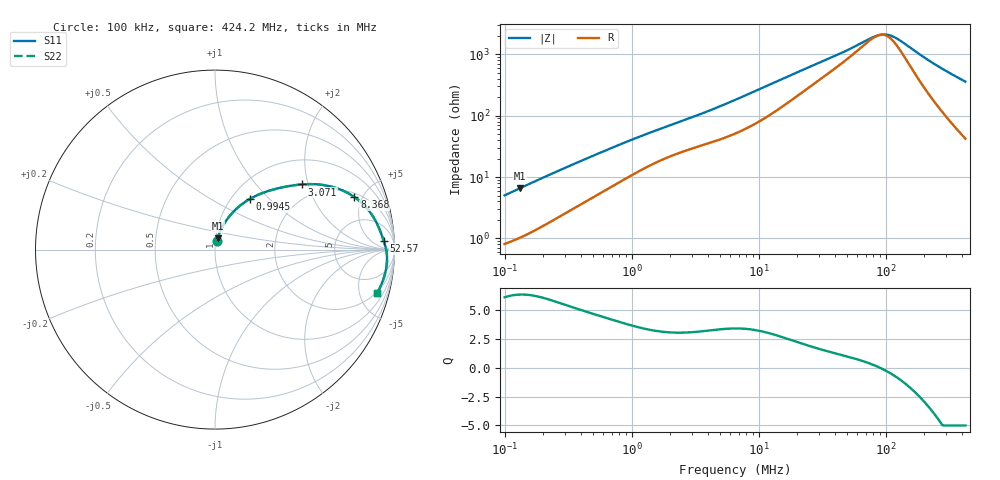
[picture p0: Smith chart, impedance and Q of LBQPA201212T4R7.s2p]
! LBQPA201212T4R7  S-PARAMETER MODEL  ( General Type )
! Model Generated by TAIYO YUDEN Corporation (http://www.ty-top.com)
! Version 1.0
! TAIYO YUDEN Control No. 191025NI43SB-FBB
! Copyright(c) 2019 TAIYO YUDEN CO.,LTD. All Rights Reserved.
! Product Description (link to TY-COMPAS)
! https://ds.yuden.co.jp/TYCOMPAS/or/detail?pn=LBQPA201212T4R7M&u=M
! Products Name : Inductors
! Characteristics :
!  Inductance : 4.7 uH , SRF(min) : 45 MHz , DC Resistance(max) : 0.65 Ohm
!  Rated Current : Saturation :360 mA , Temp Rise : 395 mA (20 degC)
!  Case Size : 2.0 x 1.25 / 0.079 x 0.049 [mm/inch] , Thickness : 1.25 / 0.049 [mm/inch]
!  (Conditions: Temperature = 25 degC , DC Bias Current/Voltage = 0A / 0V)
! External Node Assignments :
!  1  o---GGG---o  2
! GND o---------o GND
! Frequency Range : 0.1MHz  -  424.248007MHz  [ 402 STEP ]
# MHz S RI R 50
! Freq[MHz].  S11 Real  S11 Imag  S21 Real  S21 Imag  S12 Real  S12 Imag  S22 Real  S22 Imag
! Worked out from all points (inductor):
!   401 points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, 100 kHz to 424.2 MHz, reference 50 ohm
!   read as one part in series: L = 7.83 uH near 104.3 kHz
!   highest Q = 6.33 at 131.2 kHz (marker M1), where L = 7.82 uH
!   self-resonance near 89.91 MHz
!   S11 on the Smith chart (normalised r, x): 100 kHz: 1.02, +0.10; 994.5 kHz: 1.21, +0.78; 3.071 MHz: 1.59, +1.83; 8.368 MHz: 2.30, +4.33; 52.57 MHz: 19, +16; 424.2 MHz: 1.84, -7.11
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0.1  0.0105 0.0487  0.9895 -0.0487  0.9895 -0.0487  0.0105 0.0487
0.131189  0.0141 0.0629  0.9859 -0.0629  0.9859 -0.0629  0.0141 0.0629
0.245453  0.0323 0.11  0.9677 -0.11  0.9677 -0.11  0.0323 0.11
0.40516  0.064 0.1639  0.936 -0.1639  0.936 -0.1639  0.064 0.1639
0.641424  0.1164 0.2246  0.8836 -0.2246  0.8836 -0.2246  0.1164 0.2246
0.994479  0.1951 0.2826  0.8049 -0.2826  0.8049 -0.2826  0.1951 0.2826
1.641544  0.3133 0.3314  0.6867 -0.3314  0.6867 -0.3314  0.3133 0.3314
3.071313  0.4842 0.3632  0.5158 -0.3632  0.5158 -0.3632  0.4842 0.3632
4.567053  0.606 0.3594  0.394 -0.3594  0.394 -0.3594  0.606 0.3594
6.650878  0.7187 0.3259  0.2813 -0.3259  0.2813 -0.3259  0.7187 0.3259
8.368324  0.7771 0.2925  0.2229 -0.2925  0.2229 -0.2925  0.7771 0.2925
14.10473  0.8672 0.2039  0.1328 -0.2039  0.1328 -0.2039  0.8672 0.2039
26.38981  0.9157 0.1153  0.0843 -0.1153  0.0843 -0.1153  0.9157 0.1153
52.5672  0.9402 0.0483  0.0598 -0.0483  0.0598 -0.0483  0.9402 0.0483
84.97731  0.9526 0.00547  0.0474 -0.00547  0.0474 -0.00547  0.9526 0.00547
96.32018  0.955 -0.00686  0.045 0.00686  0.045 0.00686  0.955 -0.00686
106.9209  0.9566 -0.0177  0.0434 0.0177  0.0434 0.0177  0.9566 -0.0177
126.3615  0.9583 -0.0363  0.0417 0.0363  0.0417 0.0363  0.9583 -0.0363
195.9138  0.9554 -0.0945  0.0446 0.0945  0.0446 0.0945  0.9554 -0.0945
257.0175  0.9462 -0.139  0.0538 0.139  0.0538 0.139  0.9462 -0.139
351.5591  0.9244 -0.2003  0.0756 0.2003  0.0756 0.2003  0.9244 -0.2003
424.248  0.9031 -0.2425  0.0969 0.2425  0.0969 0.2425  0.9031 -0.2425
